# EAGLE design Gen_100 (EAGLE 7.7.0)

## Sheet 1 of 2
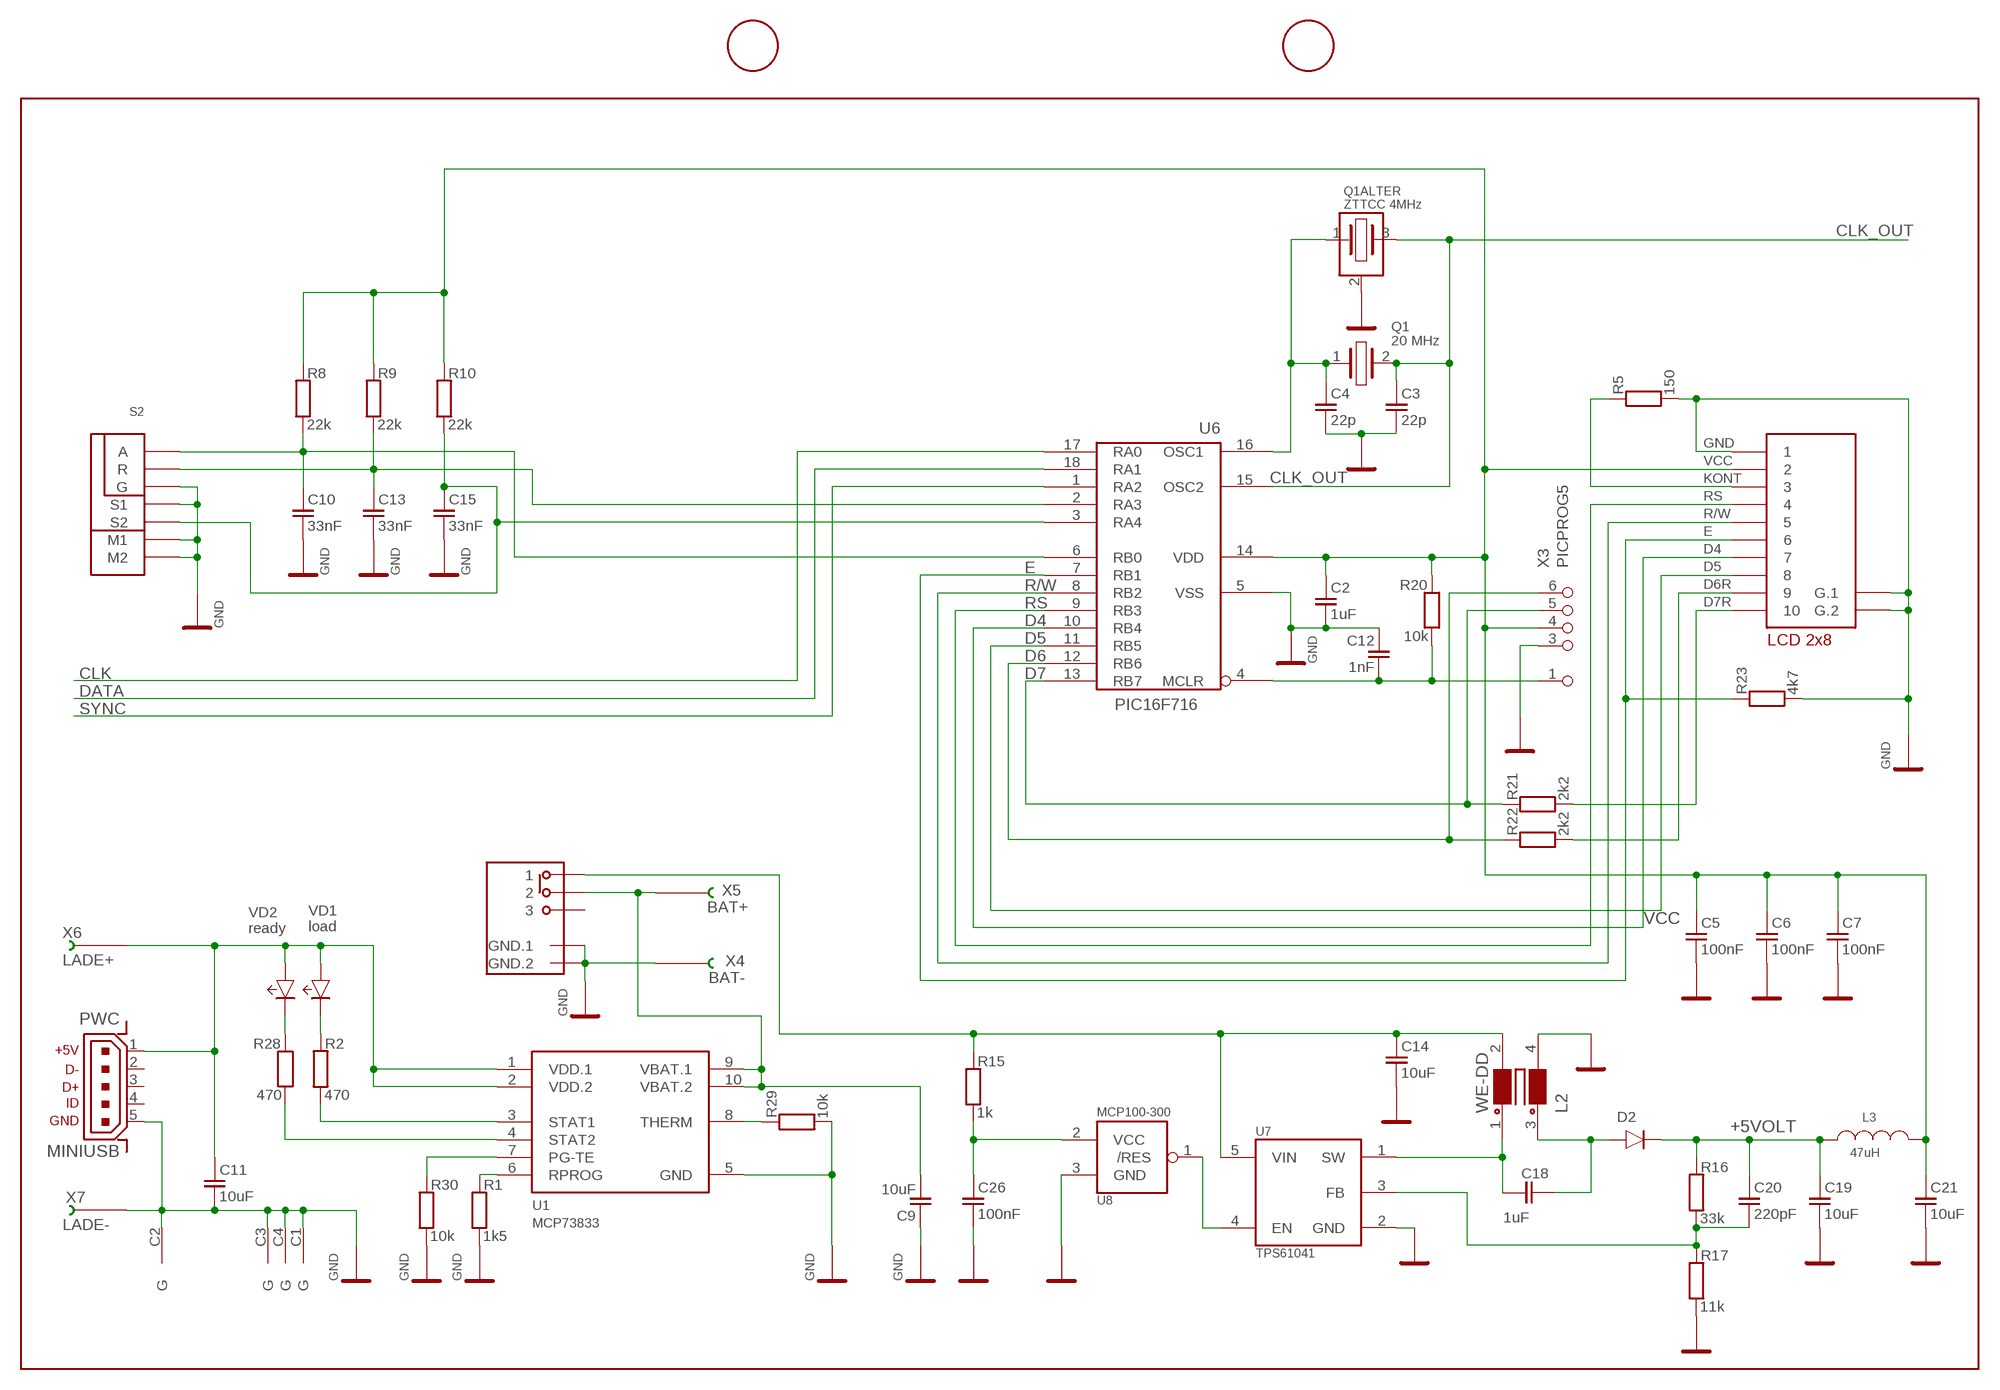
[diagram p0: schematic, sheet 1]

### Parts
C2  1uF  SMD-0603  [SOT-0603]
C3  22p  SMD-0603  [SOT-0603]
C4  22p  SMD-0603  [SOT-0603]
C5  100nF  SMD-0603  [SOT-0603]
C6  100nF  SMD-0603  [SOT-0603]
C7  100nF  SMD-0603  [SOT-0603]
C9  10uF  SMD-0805  [SOT-0805]
C10  33nF  SMD-0603  [SOT-0603]
C11  10uF  SMD-0805  [SOT-0805]
C12  1nF  SMD-0603  [SOT-0603]
C13  33nF  SMD-0603  [SOT-0603]
C14  10uF  SMD-0805  [SOT-0805]
C15  33nF  SMD-0603  [SOT-0603]
C18  1uF  SMD-0805  [SOT-0805]
C19  10uF  SMD-0805  [SOT-0805]
C20  220pF  SMD-0603  [SOT-0603]
C21  10uF  SMD-0805  [SOT-0805]
C26  100nF  SMD-0603  [SOT-0603]
D2  BAR-43  [SOT-23]
L2  WE-DD  [WE-DD_7X7]
L3  47uH  SMD-1210  [SMD-1210]
PW  MINIUSB  [UX60A-MB-5SY]
Q1  20 MHz  Q-MA306  [Q-MA306]
Q1ALTER  ZTTCC 4MHz  ZTTCC  [ZTTCC]
R1  1k5  SMD-0603  [SMD-0603]
R2  470  SMD-0603  [SMD-0603]
R5  150  SMD-0603  [SMD-0603]
R8  22k  SMD-0603  [SMD-0603]
R9  22k  SMD-0603  [SMD-0603]
R10  22k  SMD-0603  [SMD-0603]
R15  1k  SMD-0603  [SMD-0603]
R16  33k  SMD-0603  [SMD-0603]
R17  11k  SMD-0603  [SMD-0603]
R20  10k  SMD-0603  [SMD-0603]
R21  2k2  SMD-0603  [SMD-0603]
R22  2k2  SMD-0603  [SMD-0603]
R23  4k7  SMD-0603  [SMD-0603]
R28  470  SMD-0603  [SMD-0603]
R29  10k  SMD-0603  [SMD-0603]
R30  10k  SMD-0603  [SMD-0603]
S1  FAR120-1431  SXUM-1X3  [SXUM1X3]
S2  DREHGEBER-ALPS5  [DG-ALPS-ST5]
U1  MCP73833  [MSOP10-0.5]
U6  PIC16F716  PIC16F627  [SO-18L]
U7  TPS61041  [SOT23-5]
U8  MCP100-300  TC1275  [SOT23]
VD1  load  LED-SMD  [LED0805]
VD2  ready  LED-SMD  [LED0805]
X2  FP10-1UPPE  [FPC10-1U]
X3  PICPROG5  [PICPROG5]
X4  BAT-  LÖTÖSEQ  [LÖTÖSEQ]
X5  BAT+  LÖTÖSEQ  [LÖTÖSEQ]
X6  LADE+  LÖTÖSEQ  [LÖTÖSEQ]
X7  LADE-  LÖTÖSEQ  [LÖTÖSEQ]

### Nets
+5VOLT: C19.2 C20.2 D2.3(K) L3.1 R16.2
CLK: U6.17(RA0) ; also sheet 2
CLK_OUT: C3.2 Q1.2 Q1ALTER.3 U6.15(OSC2) ; also sheet 2
D4: U6.10(RB4) X2.7
D5: U6.11(RB5) X2.8
D6: R22.2 U6.12(RB6) X3.6
D6R: R22.1 X2.9
D7: R21.2 U6.13(RB7) X3.5
D7R: R21.1 X2.10
DATA: U6.18(RA1) ; also sheet 2
E: R23.2 U6.7(RB1) X2.6
GND: C2.1 C3.1 C4.1 C5.1 C6.1 C7.1 C9.2 C10.1 C11.1 C12.2 C13.1 C14.1 C15.1 C19.1 C21.1 C26.1 L2.4 PW.5 PW.C1(G) PW.C2(G) PW.C3(G) PW.C4(G) Q1ALTER.2 R1.1 R5.1 R17.1 R23.1 R29.1 R30.1 S1.GND.1 S1.GND.2 S2.G S2.M1 S2.M2 S2.S1 U1.5(GND) U6.5(VSS) U7.2(GND) U8.3(GND) X2.1 X2.P$1(G.1) X2.P$2(G.2) X3.3 X4.1 X7.1 ; also sheet 2
KONT: R5.2 X2.3
MCLR_VPP: C12.1 R20.1 U6.4(MCLR) X3.1
N$1: R2.2 VD1.K
N$2: C11.2 PW.1 U1.1(VDD.1) U1.2(VDD.2) VD1.A VD2.A X6.1
N$3: R28.2 VD2.K
N$5: C4.2 Q1.1 Q1ALTER.1 U6.16(OSC1)
N$7: R2.1 U1.3(STAT1)
N$8: R28.1 U1.4(STAT2)
N$9: C9.1 S1.2 U1.9(VBAT.1) U1.10(VBAT.2) X5.1
N$10: R30.2 U1.7(PG-TE)
N$11: R1.2 U1.6(RPROG)
N$12: R29.2 U1.8(THERM)
N$15: U7.4(EN) U8.1(/RES)
N$17: C26.2 R15.1 U8.2(VCC)
N$19: C14.2 L2.2 R15.2 S1.1 U7.5(VIN)
N$20: C18.2 L2.1 U7.1(SW)
N$22: C10.2 R8.1 S2.A U6.6(RB0)
N$23: C13.2 R9.1 S2.R U6.2(RA3)
N$24: C15.2 R10.1 S2.S2 U6.3(RA4)
N$25: C18.1 D2.1(A) L2.3
N$27: C20.1 R16.1 R17.2 U7.3(FB)
R/W: U6.8(RB2) X2.5
RS: U6.9(RB3) X2.4
SYNC: U6.1(RA2) ; also sheet 2
VCC: C2.2 C5.2 C6.2 C7.2 C21.2 L3.2 R8.2 R9.2 R10.2 R20.2 U6.14(VDD) X2.2 X3.4 ; also sheet 2
Unconnected: PW.2 PW.3 PW.4 S1.3

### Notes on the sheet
- LCD 2x8

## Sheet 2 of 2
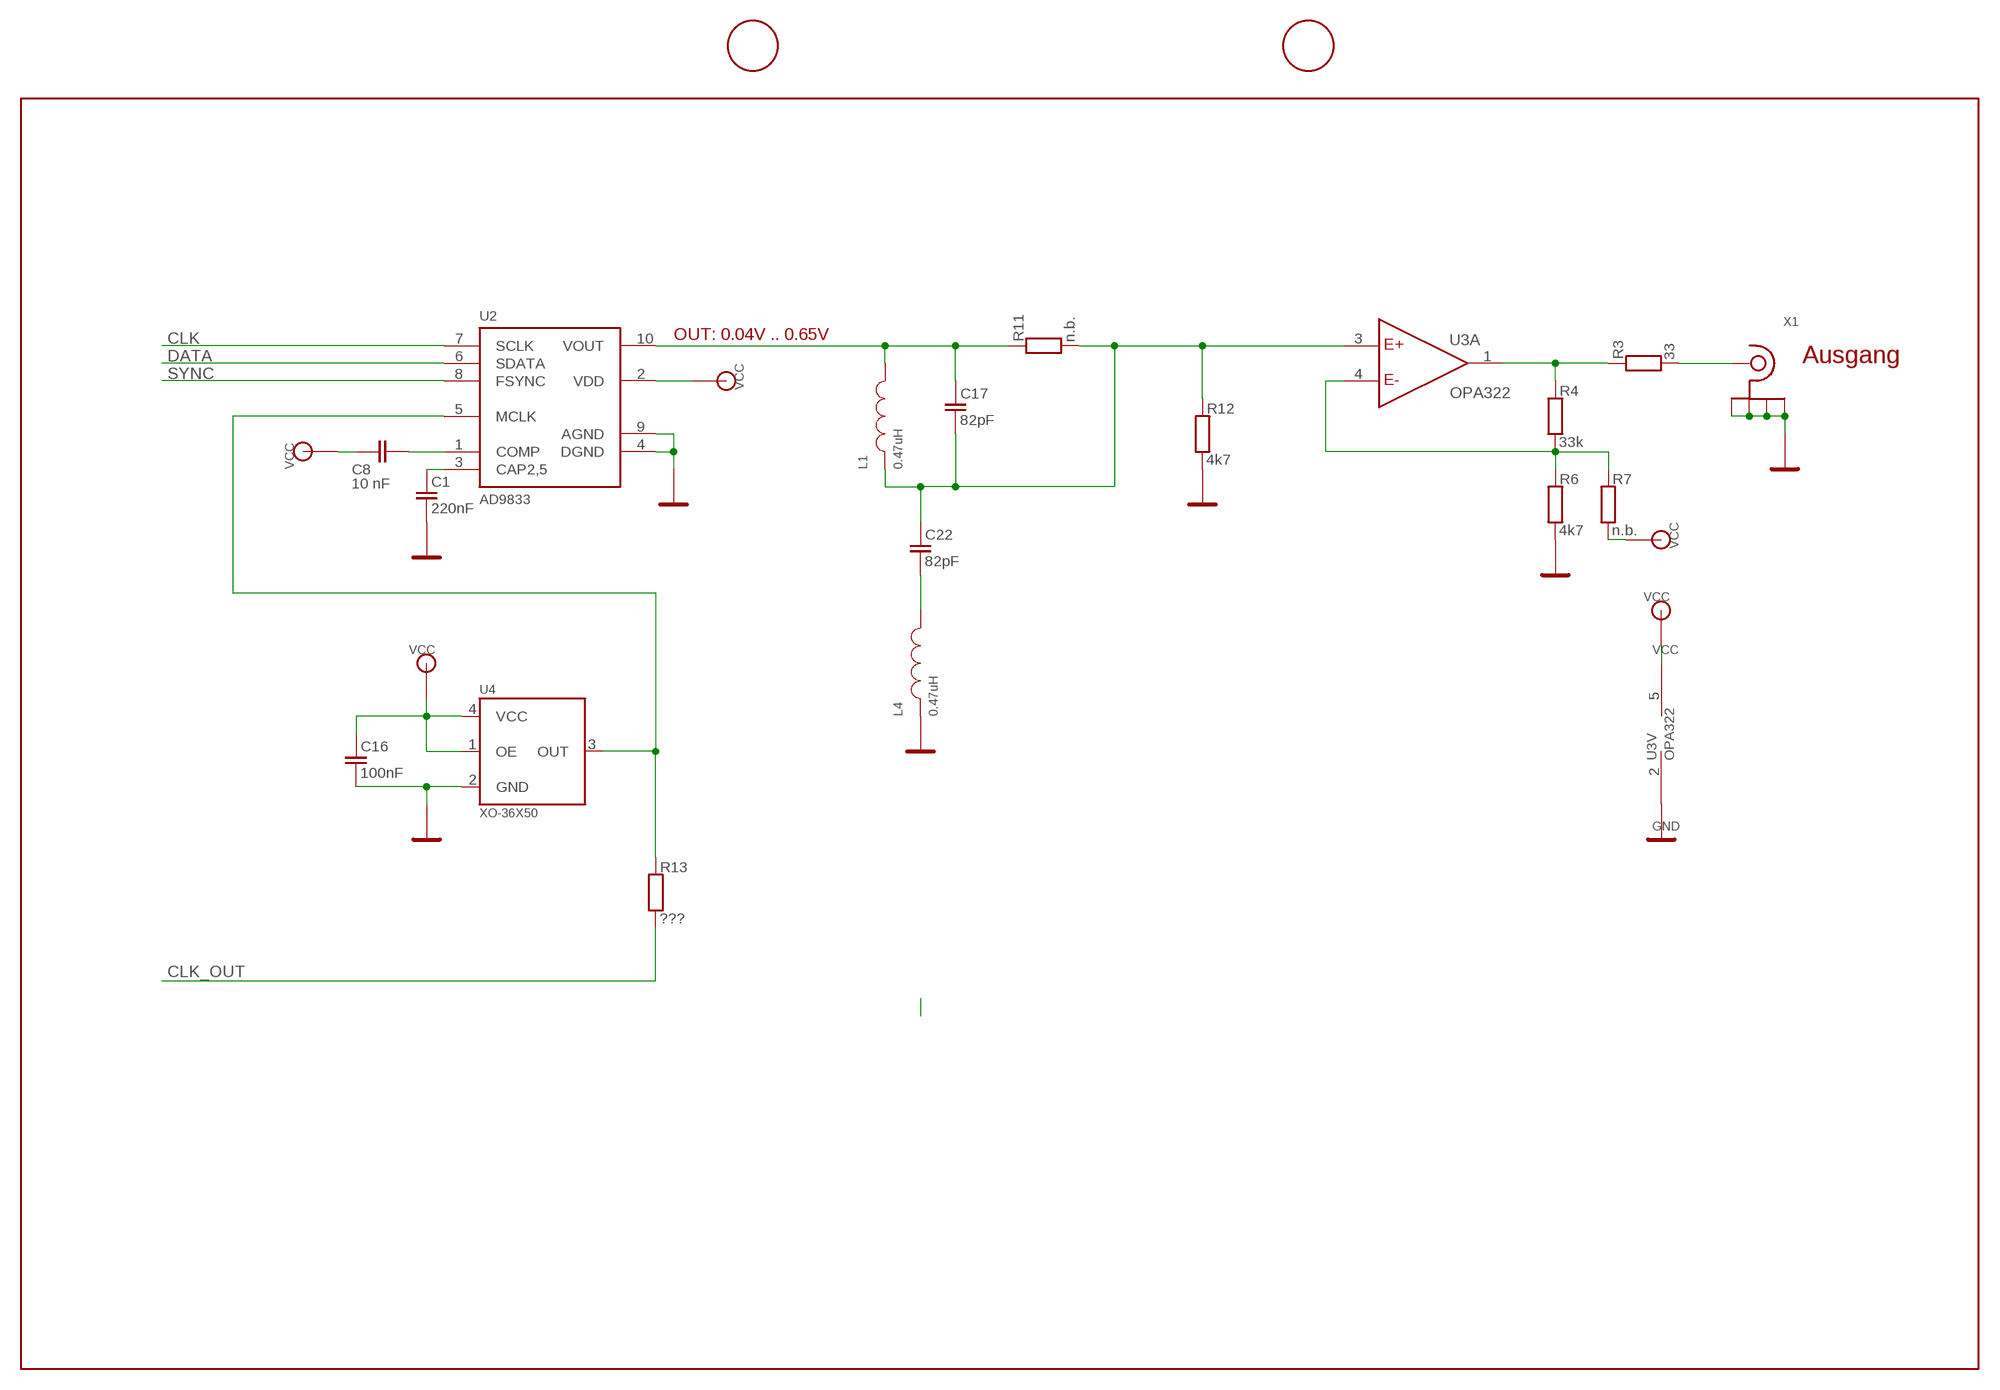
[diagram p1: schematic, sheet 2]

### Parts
C1  220nF  SMD-0603  [SOT-0603]
C8  10 nF  SMD-0603  [SOT-0603]
C16  100nF  SMD-0603  [SOT-0603]
C17  82pF  SMD-0603  [SOT-0603]
C22  82pF  SMD-0603  [SOT-0603]
L1  0.47uH  SMDL-0805  [SMDL-0805]
L4  0.47uH  SMDL-0805  [SMDL-0805]
R3  33  SMD-0805  [SMD-0805]
R4  33k  SMD-0603  [SMD-0603]
R6  4k7  SMD-0603  [SMD-0603]
R7  n.b.  SMD-0603  [SMD-0603]
R11  n.b.  SMD-0603  [SMD-0603]
R12  4k7  SMD-0603  [SMD-0603]
R13  ???  SMD-0603  [SMD-0603]
U2  AD9833  [RM-10]
U3  OPA322  [SOT23-5]
U4  XO-36X50  [XO-36X50]
X1  SMA-EDGE  [SMA-EDGE]

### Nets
CLK: U2.7(SCLK) ; also sheet 1
CLK_OUT: R13.1 ; also sheet 1
DATA: U2.6(SDATA) ; also sheet 1
GND: C1.1 C16.1 L4.1 R6.1 R12.1 U2.4(DGND) U2.9(AGND) U3.2(V:GND) U4.2(GND) X1.GND@1(GND) X1.GND@2(GND) X1.GND@3(GND) X1.GND@4(GND) ; also sheet 1
N$6: R3.2 R4.2 U3.1(A:O)
N$13: R3.1 X1.A
N$14: C17.2 L1.2 R11.2 U2.10(VOUT)
N$16: C1.2 U2.3(CAP2,5)
N$18: C8.1 U2.1(COMP)
N$21: R4.1 R6.2 R7.2 U3.4(A:E-)
N$28: R13.2 U2.5(MCLK) U4.3(OUT)
N$29: C17.1 C22.2 L1.1 R11.1 R12.2 U3.3(A:E+)
N$31: C22.1 L4.2
SYNC: U2.8(FSYNC) ; also sheet 1
VCC: C8.2 C16.2 R7.1 U2.2(VDD) U3.5(V:VCC) U4.1(OE) U4.4(VCC) ; also sheet 1

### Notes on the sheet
- OUT: 0.04V .. 0.65V
- Ausgang

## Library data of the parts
C1-C8 C10 C12 C13 C15-C17 C20 C22 C26 = C_KERAM:SMD-0603
C9 C11 C14 C18 C19 C21 = C_KERAM:SMD-0805
D2 = DIODEN:BAR-43
L1 L4 = L:SMDL-0805
L2 = L:WE-DD
L3 = L:SMD-1210
PW = mini-usb:MINIUSB
Q1 = Z_SPECIA:Q-MA306
Q1ALTER = Z_SPECIA:ZTTCC
R1 R2 R4-R13 R15-R17 R20-R23 R28-R30 = R:SMD-0603
R3 = R:SMD-0805
S1 = HAMRAD:SXUM-1X3
S2 = HAMRAD:DREHGEBER-ALPS5: Drehgeber von ALPS mit Taster, alle Wechsel zwischen den Rastunngen
U1 = MIC_CHIP:MCP73833
U2 = ANALOG_D:AD9833
U3 = TI_OPV:OPA322
U4 = Z_SPECIA:XO-36X50: MEMS Oszillator, programmierbar, 5x3.6
U6 = MIC_CHIP:PIC16F627
U7 = TI:TPS61041
U8 = MIC_CHIP:TC1275
VD1 VD2 = DIODEN:LED-SMD
X1 = HAMRAD:SMA-EDGE
X2 = Z_CONNEC:FP10-1UPPE
X3 = PINHD-Q:PICPROG5
X4-X7 = Z_CONNEC:LÖTÖSEQ

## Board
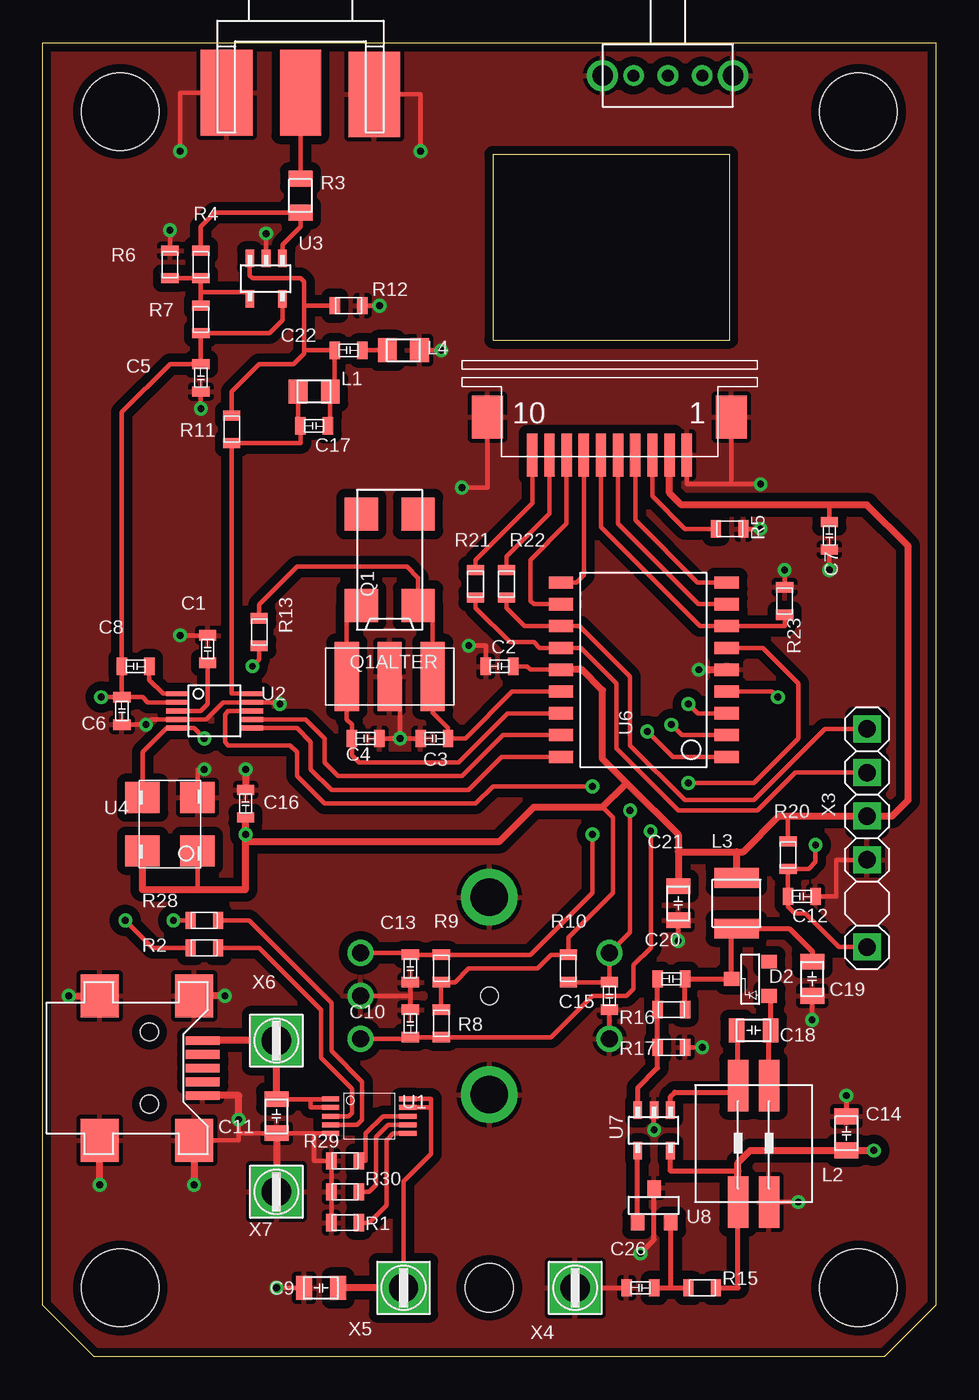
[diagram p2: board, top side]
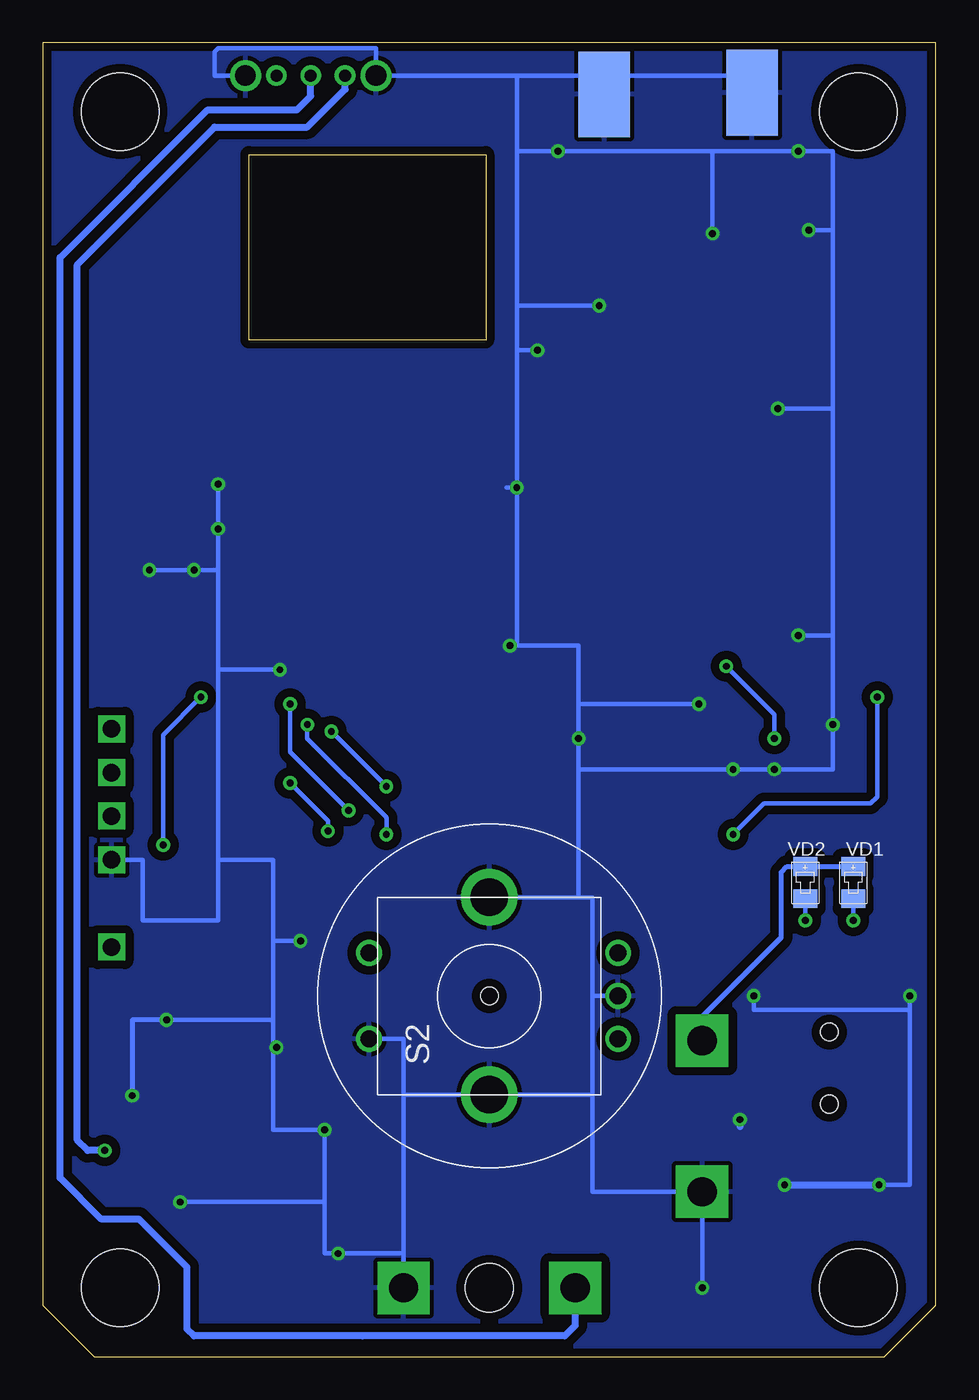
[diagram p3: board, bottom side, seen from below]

Size 52 x 76.5 mm. Coordinates in mm from the lower left corner, seen from the top.
Outline: 26.2,70 26.2,59.2 40,59.2 40,70 26.2,70
Copper layers (1*16): Top 0.035mm / dielectric 1.5mm / Bottom 0.035mm
Design rules "default *": minimum track width 0.15mm, minimum drill 0.3mm, track to track 0.15mm, track to pad 0.15mm, pad to pad 0.15mm, via to via 0.15mm, smd to smd 0mil, copper to edge 0.15mm, drill to drill 0.15mm, minimum pad ring 0.15mm, minimum via ring 0.15mm, stop-mask expansion 4mil, vias tented up to drill 0mil, thermal gap 10mil
Holes 2.8 mm at 26,4
Holes 1 mm at 26,21

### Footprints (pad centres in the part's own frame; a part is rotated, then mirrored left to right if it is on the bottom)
SOT-0603 = smd 0.6 x 1: 1 -0.8,0; 2 0.8,0
SOT-0805 = smd 0.914 x 1.397: 1 -0.991,0; 2 0.991,0
SOT-23 = smd 0.8 x 0.9: 1 -1,-1.1; 2 1,-1.1; 3 0,1.1
SMDL-0805 = smd 1.092 x 1.397: 1 -0.94,0; 2 0.94,0
WE-DD_7X7 = smd 1.2 x 3: 1 0.91,-3.39; 2 0.91,3.41; 3 -0.89,-3.39; 4 -0.89,3.41
SMD-1210 = smd 1.143 x 2.591: 1 -1.473,0; 2 1.473,0
UX60A-MB-5SY = smd 0.5 x 2: 1 -1.6,3.1; 2 -0.8,3.1; 3 0,3.1; 4 0.8,3.1; 5 1.6,3.1 | smd 2.5 x 2.2: C1 -4.2,2.6; C2 -4.2,-2.9; C3 4.2,-2.9; C4 4.2,2.6 | hole 1.016: -2.1,0; 2.1,0
Q-MA306 = smd 1.93 x 1.93: 1 -2.667,1.651; 2 -2.667,-1.651; 3 2.667,-1.651; 4 2.667,1.651
ZTTCC = smd 1.4 x 4: 1 -2.5,0; 2 0,0; 3 2.5,0
SMD-0603 = smd 0.6 x 1: 1 -0.8,0; 2 0.8,0
SMD-0805 = smd 0.914 x 1.397: 1 -0.991,0; 2 0.991,0
SXUM1X3 = drill 0.7 pad 1.2: 1 -2,0; 2 0,0; 3 2,0 | drill 1.2 pad 1.7: GND.1 -3.8,0; GND.2 3.8,0
DG-ALPS-ST5 = drill 1: A -2.5,-7.5; G 0,-7.5; R 2.5,-7.5; S1 -2.5,7; S2 2.5,7 | drill 2.2: M1 -5.75,0; M2 5.75,0
MSOP10-0.5 = smd 1 x 0.29: 1 -2.25,1; 2 -2.25,0.5; 3 -2.25,0; 4 -2.25,-0.5; 5 -2.25,-1; 6 2.25,-1; 7 2.25,-0.5; 8 2.25,0; 9 2.25,0.5; 10 2.25,1
RM-10 = smd 0.279 x 1.27: 1 -1,-2.2; 2 -0.5,-2.2; 3 0,-2.2; 4 0.5,-2.2; 5 1,-2.2; 6 1,2.2; 7 0.5,2.2; 8 0,2.2; 9 -0.5,2.2; 10 -1,2.2
SOT23-5 = smd 0.508 x 1.016: 1 -0.953,-1.143; 2 0,-1.143; 3 0.953,-1.143; 4 0.953,1.206; 5 -0.953,1.206
XO-36X50 = smd 1.8 x 2: 1 -1.55,-1.6; 2 1.55,-1.6; 3 1.55,1.6; 4 -1.55,1.6
SO-18L = smd 0.711 x 1.422: 1 -5.08,-4.826; 2 -3.81,-4.826; 3 -2.54,-4.826; 4 -1.27,-4.826; 5 0,-4.826; 6 1.27,-4.826; 7 2.54,-4.826; 8 3.81,-4.826; 9 5.08,-4.826; 10 5.08,4.826; 11 3.81,4.826; 12 2.54,4.826; 13 1.27,4.826; 14 0,4.826; 15 -1.27,4.826; 16 -2.54,4.826; 17 -3.81,4.826; 18 -5.08,4.826
SOT23-5' = smd 1.016 x 0.508: 1 -1.143,0.953; 2 -1.143,0; 3 -1.143,-0.953; 4 1.206,-0.953; 5 1.206,0.953
SOT23 = smd 0.889 x 0.787: 1 -1.016,0.965; 2 -1.016,-0.965; 3 1.016,0
ABS-100 = hole 4.5: -21.5,68.5; 21.5,68.5; -21.5,0; 21.5,0
LED0805 = smd 1.092 x 1.397: A 0.94,0; K -0.94,0
SMA-EDGE = smd 5 x 2.4: A 0,0 | smd 5 x 3: GND@1 0,4.3; GND@2 -0.1,-4.3 | smd 5 x 3 bottom: GND@3 0,4.3; GND@4 -0.1,-4.3
FPC10-1U = smd 0.6 x 2.5: 1 -4.5,1.5; 2 -3.5,1.5; 3 -2.5,1.5; 4 -1.5,1.5; 5 -0.5,1.5; 6 0.5,1.5; 7 1.5,1.5; 8 2.5,1.5; 9 3.5,1.5; 10 4.5,1.5 | smd 1.8 x 2.5: P$1 7.1,-0.7; P$2 -7.1,-0.7
PICPROG5 = drill 1.016 pad 1.575 square: 1 -6.35,0; 3 -1.27,0; 4 1.27,0; 5 3.81,0; 6 6.35,0
LÖTÖSEQ = drill 1.702 pad 3.048 square: 1 0,0

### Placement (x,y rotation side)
C1  9.6,41.2 270 top
C2  26.6,40.2 0 top
C3  22.8,36 0 top
C4  18.8,36 180 top
C5  9.2,57 90 top
C6  4.6,37.6 90 top
C7  45.8,47.8 90 top
C8  5.4,40.2 180 top
C9  16.2,4 180 top
C10  21.4,19.4 270 top
C11  13.6,14 90 top
C12  44.2,26.8 0 top
C13  21.4,22.6 90 top
C14  46.8,13 270 top
C15  33,21 90 top
C16  11.8,32.2 270 top
C17  15.8,54.2 180 top
C18  41.4,19 180 top
C19  44.8,22 90 top
C20  36.6,22 0 top
C21  37,26.4 90 top
C22  17.8,58.6 180 top
C26  34.8,4 0 top
D2  41.2,22 90 top
L1  15.8,56.2 180 top
L2  41.4,12.4 180 top
L3  40.4,26.4 90 top
L4  21,58.6 180 top
PW  6.2,16.8 270 top
Q1  20.2,46.4 90 top
Q1ALTER  20.2,39.6 0 top
R1  17.6,7.8 0 top
R2  9.4,23.8 180 top
R3  15,67.6 270 top
R4  9.2,63.6 90 top
R5  40,48.2 180 top
R6  7.4,63.6 270 top
R7  9.2,60.4 90 top
R8  23.2,19.4 90 top
R9  23.2,22.6 270 top
R10  30.6,22.6 90 top
R11  11,54 270 top
R12  17.8,61.2 180 top
R13  12.6,42.2 270 top
R15  38.4,4 0 top
R16  36.6,20.2 0 top
R17  36.6,18 180 top
R20  43.4,29.2 90 top
R21  25.2,45 270 top
R22  27,45 270 top
R23  43.2,44 270 top
R28  9.4,25.4 180 top
R29  17.6,11.4 0 top
R30  17.6,9.6 0 top
S1  36.4,74.6 0 top
S2  26,21 90 bottom
U1  19,14 0 top
U2  10,37.6 270 top
U3  13,62.8 180 top
U4  7.4,31 90 top
U6  35,40 90 top
U7  TPS61041  [SOT23-5']  35.6,13.2 270 top
U8  35.6,8.8 90 top
U$13  [ABS-100]  26,4 0 bottom
VD1  4.8,27.6 90 bottom
VD2  7.6,27.6 90 bottom
X1  15,73.6 90 top
X2  33,54 180 top
X3  48,30.2 90 top
X4  31,4 0 top
X5  21,4 0 top
X6  13.6,18.4 0 top
X7  13.6,9.6 0 top

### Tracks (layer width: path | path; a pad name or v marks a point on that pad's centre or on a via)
+5VOLT
  Top 0.3: 40.1,24.93 D2.3 C20.2 R16.2 | C19.2 44.8,23.6 43.47,24.93 L3.1
  Top 0.4: 40.1,24.93 L3.1
CLK
  Top 0.25: U6.17 26.79,36.19 24.4,33.8 17.2,33.8 16.4,34.6 16.4,36 15.3,37.1 U2.7
CLK_OUT
  Top 0.25: U6.15 27.33,38.73 24.6,36 C3.2 23.6,36.6 22.7,37.5 Q1ALTER.3 22.7,43.73 Q1.2 21.85,45.35 21.2,46 14.8,46 12.6,43.8 R13.1
D4
  Top 0.25: X2.7 31.5,45.5 31.08,45.08 U6.10
D5
  Top 0.25: X2.8 30.5,48.5 28.4,46.4 28.4,44 28.59,43.81 U6.11
D6
  Top 0.25: X3.6 45.55,36.55 41.4,32.4 37.4,32.4 34.2,35.6 34.2,36.6 34.2,39.6 31.26,42.54 U6.12 28.06,42.54 27,43.6 R22.2
D6R
  Top 0.25: X2.9 29.5,49.1 27,46.6 R22.1
D7
  Top 0.25: X3.5 43.81,34.01 41.6,31.8 37,31.8 33.4,35.4 33.4,37.2 33.4,38.6 33.4,39.2 31.33,41.27 U6.13 28.93,41.27 28.6,41.6 27.2,41.6 25.2,43.6 R21.2
D7R
  Top 0.25: X2.10 28.5,49.7 25.2,46.4 R21.1
DATA
  Top 0.25: U6.18 26.72,34.92 24.8,33 16.8,33 15.6,34.2 15.6,35.8 14.8,36.6 U2.6
E
  Top 0.25: X2.6 32.5,48.3 38.26,42.54 U6.7 43.2,42.54 R23.2
GND  (via drill 0.4 pad 0.8)
  Top 0.25: X2.P$1 25.9,50.6 v24.4,50.6 | 40.1,50.8 X2.P$2 | v41.8,50.8 40.1,50.8 | U1.5 15.8,13.01 | 15.8,13.01 C11.1 11.4,13.01 | 11.4,13.01 v11.4,13.8 | PW.C4 11.4,12.6 11.4,13.01 | v13.6,4 C9.2 | 15.8,13.01 15.8,11.4 R29.1 R30.1 R1.1 | L2.4 v44,9 | v37,24.2 C21.1 | v38.4,18 R17.1 | 21.4,21 C13.1 | S2.G 21.4,21 | 21.4,21 C10.1 | X2.1 37.5,50.8 40.1,50.8 | C12.2 46.2,26.8 46.2,28.93 X3.3 | v41.8,48.2 R5.1 | C2.1 25.8,41.4 v24.8,41.4 | v43.2,45.8 R23.1 | S2.S1 C15.1 | v13.8,38 13.7,38.1 U2.9 10.5,38.1 9.5,37.1 U2.4 6.3,37.1 v6,36.8 C6.1 | U4.2 9,34.2 v9.4,34.2 | v8,42 C1.1 | v45.8,45.8 C7.1 | X1.GND@3 8,73.6 v8,70.2 | v13,65.4 U3.2 | v7.4,65.6 R6.1 | v9.2,55.2 C5.1 | v19.6,61.2 R12.1 | v23.2,58.6 L4.1 | v20.8,36 C3.1 | v20.8,36 C4.1 | Q1ALTER.2 20.8,39.6 v20.8,36 | X1.GND@4 22,73.5 v22,70.2
  Top 0.3: X4.1 C26.1 | U8.3 35.6,6.8 v34.8,6 | v35.6,13.2 U7.2 | v44.8,19.6 C19.1 | v46.8,15.2 C14.1
  Top 0.4: C11.1 X7.1 | v3.3,10 PW.C3 | PW.C4 v8.8,10 | PW.5 11.4,15.2 v11.4,13.8 | v1.5,21 PW.C2 | v10.6,21 PW.C1 | v38.2,40 U6.5 | v11.8,34.2 C16.1
  Bottom 0.25: v24.4,50.6 25,50.6 | v13.6,4 X7.1 20,9.6 20,15.25 | 31,6 v34.8,6 35.6,6 35.6,9 | 31,6 X4.1 | 35.6,9 v35.6,13.2 38.6,13.2 38.6,18 | 35.6,9 v44,9 | 31,15.25 S2.M1 20,15.25 | 31,15.25 31,6 | 38.6,24.2 v37,24.2 | 38.6,18 38.6,19.6 | 38.6,19.6 38.6,24.2 | 38.6,19.6 v44.8,19.6 | 41.8,28.93 41.8,25.4 46.2,25.4 46.2,28.93 X3.3 | 38.6,24.2 38.6,28.93 41.8,28.93 | 38.6,18 v38.4,18 | 20,15.25 20,21 | 20,21 S2.G | 20.8,26.75 20,26.75 20,21 | 20.8,26.75 S2.M2 | 20.8,26.75 20.8,34.2 | 41.8,28.93 41.8,40 | v41.8,50.8 v41.8,48.2 41.8,45.8 | 41.8,40 v38.2,40 | 41.8,40 41.8,45.8 | v24.4,50.6 24.4,41.4 v24.8,41.4 20.8,41.4 20.8,38 | 41.8,45.8 v43.2,45.8 v45.8,45.8 | S2.S1 31,18.5 31,15.25 | 20.8,34.2 v20.8,36 20.8,38 | 20.8,38 v13.8,38 | 20.8,34.2 v11.8,34.2 v9.4,34.2 6,34.2 v6,36.8 6,42 | 6,42 v8,42 | X1.GND@3 10.7,74.6 19.3,74.6 | v24.4,50.6 24.4,57 | 24.4,61.2 24.4,58.6 | 24.4,70.2 24.4,61.2 | 6,42 6,55.2 | 6,55.2 6,65.6 | 6,65.6 6,70.2 v8,70.2 13,70.2 | 13,70.2 v22,70.2 24.4,70.2 | 20.4,74.6 19.3,74.6 | 19.3,74.6 X1.GND@4 20.4,74.6 | 13,70.2 v13,65.4 | 6,65.6 v7.4,65.6 | 6,55.2 v9.2,55.2 | S1.GND.2 42,74.6 42,76 41.8,76.2 32.6,76.2 S1.GND.1 24.4,74.6 | 1.5,20.2 v1.5,21 | 1.5,20.2 10.6,20.2 v10.6,21 | v3.3,10 1.5,10 1.5,20.2 | 24.4,61.2 v19.6,61.2 | 24.4,58.6 24.4,47.4 | 24.4,58.6 v23.2,58.6 | 24.4,74.6 20.4,74.6 | 24.4,70.2 24.4,74.6
  Bottom 0.3: v46.8,15.2 46.8,19.6 v44.8,19.6
  Bottom 0.4: v8.8,10 v3.3,10 | v11.4,13.8 11.4,13.4
  pour Bottom (isolate 0.5): 0.4,76 0.4,3 3,0.4 49,0.4 51.6,3 51.6,76
  pour Top (isolate 0.5): 0.6,76 0.4,3.4 3.4,0.4 48.8,0.4 51.6,3.2 51.6,76.2
KONT
  Top 0.25: X2.3 35.5,50.1 37.4,48.2 R5.2
MCLR_VPP  (via drill 0.4 pad 0.8)
  Top 0.25: U6.4 42.47,38.73 v42.8,38.4 | v45,29.8 45,28.8 44.6,28.4 R20.1 C12.1 43.4,26.2 43.8,25.8 44.4,25.8 46.35,23.85 X3.1
  Bottom 0.25: v45,29.8 45,35.2 45,36.2 v42.8,38.4
N$1  (via drill 0.4 pad 0.8)
  Top 0.25: v4.8,25.4 6.4,23.8 R2.2
  Bottom 0.25: VD1.K v4.8,25.4
N$2
  Top 0.25: C11.2 15.6,14.99 | 15.6,14.99 U1.1 | U1.2 15.6,14.5 15.6,14.99
  Top 0.4: PW.1 X6.1 C11.2
  Bottom 0.3: VD1.A VD2.A 8.66,28.54 9,28.2 9,24.4 13.6,19.8 13.6,19.2 X6.1
N$3  (via drill 0.4 pad 0.8)
  Top 0.25: v7.6,25.4 R28.2
  Bottom 0.25: VD2.K v7.6,25.4
N$5
  Top 0.25: U6.16 27.06,37.46 24.2,34.6 18.4,34.6 18,35 C4.2 18,36.8 17.7,37.1 Q1ALTER.1 17.7,43.73 Q1.1
N$6
  Top 0.25: U3.1 13.95,64.75 15,65.8 R3.2 10.01,66.61 9.2,65.8 R4.2
N$7
  Top 0.25: U1.3 17.8,14 18,14.2 18,15.6 16.2,17.4 16.2,20.2 12.6,23.8 R2.1
N$8
  Top 0.25: U1.4 18.3,13.5 18.6,13.8 18.6,16 16.8,17.8 16.8,20.6 12,25.4 R28.1
N$9
  Top 0.25: X5.1 21,10.2 22.6,11.8 22.6,14.4 | 22.6,14.4 22.6,15 U1.10 | U1.9 22.5,14.5 22.6,14.4
  Top 0.4: X5.1 C9.1
  Bottom 0.4: S1.2 36.4,73.4 37.2,72.6 42.4,72.6 51,64 51,10.4 48.6,8 46.4,8 43.6,5.2 43.6,1.6 43.2,1.2 33.4,1.2 21.6,1.2 21,1.8 X5.1
N$10
  Top 0.25: U1.7 20.1,13.5 19.4,12.8 19.4,10 19,9.6 R30.2
N$11
  Top 0.25: U1.6 20.4,13 20,12.6 20,8.8 19,7.8 R1.2
N$12
  Top 0.25: U1.8 19.8,14 18.8,13 18.8,11.4 R29.2
N$13
  Top 0.25: R3.1 X1.A
N$14
  Top 0.25: U2.10 11,38.6 R11.2 15,53.2 C17.2 14.86,54.2 L1.2
N$15
  Top 0.3: U8.1 34.63,11.99
  Top 0.4: 34.63,11.99 U7.4
N$16
  Top 0.25: U2.3 9.2,37.6 9.6,38 C1.2
N$17
  Top 0.3: 36.56,4 U8.2 | C26.2 36.56,4 | 36.56,4 R15.1
N$18
  Top 0.25: U2.1 7,38.6 6.2,39.4 C8.1
N$19  (via drill 0.4 pad 0.8)
  Top 0.3: U7.5 36.55,10.8 40.49,10.8 | C14.2 | L2.2 40.49,4 R15.2
  Top 0.4: v48.4,12 C14.2 41.2,12 40.49,11.29 40.49,10.8 L2.2
  Bottom 0.4: S1.1 34.4,73.8 36.6,71.6 42,71.6 50,63.6 50,12.6 49.4,12 v48.4,12
N$20
  Top 0.3: C18.2 40.49,19 L2.1 40.49,15.4 36.8,15.4 36.55,15.15 U7.1
N$21
  Top 0.25: R6.2 R4.1 9.2,62 | U3.4 12.05,62 9.2,62 | R7.2 9.2,62
N$22  (via drill 0.4 pad 0.8)
  Top 0.25: S2.A 21.4,18.5 C10.2 R8.1 29.6,18.6 32,21 34,21 34.4,21.4 34.4,22.8 35.4,23.8 v35.4,30.6 | U6.6 41.93,41.27 44,39.2 44,36 41.4,33.4 v37.6,33.4
  Bottom 0.25: v37.6,33.4 35.4,31.2 v35.4,30.6
N$23  (via drill 0.4 pad 0.8)
  Top 0.25: S2.R 21.4,23.5 C13.2 R9.1 28.4,23.4 32,27 v32,30.4 | U6.2 37.21,36.19 v36.6,36.8
  Bottom 0.25: v36.6,36.8 36.6,36 32,31.4 32,31 v32,30.4
N$24  (via drill 0.4 pad 0.8)
  Top 0.25: U6.3 38.14,37.46 v37.6,38 | v34.2,31.8 34.2,24.7 S2.S2 C15.2 R10.1
  Bottom 0.25: v37.6,38 37.6,35.2 v34.2,31.8
N$25
  Top 0.3: 42.39,21 C18.1 42.29,19 L2.3
  Top 0.4: 42.39,21 D2.1
N$27
  Top 0.3: C20.1 R16.1 R17.2 35.8,16.8 34.65,15.65 U7.3
N$28  (via drill 0.4 pad 0.8)
  Top 0.25: U4.3 5.8,35.2 7.2,36.6 U2.5 8.8,36.6 v9.4,36 | v12.2,40.2 12.6,40.6 R13.2
  Bottom 0.25: v9.4,36 9.4,37.4 v12.2,40.2
N$29
  Top 0.25: U3.3 12.05,62.95 12.2,62.8 15,62.8 15.2,62.6 15.2,61.2 | 15.2,58.6 15.2,58.4 14.6,57.8 12.6,57.8 11,56.2 R11.1 | 15.2,58.6 15.2,61.2 | 15.2,61.2 R12.2 | 15.2,58.6 C22.2 17,56.2 L1.1 16.74,54.2 C17.1
N$31
  Top 0.25: L4.2 C22.1
R/W
  Top 0.25: X2.5 33.5,48.5 38.19,43.81 U6.8
RS
  Top 0.25: X2.4 34.5,48.7 38.12,45.08 U6.9
SYNC  (via drill 0.4 pad 0.8)
  Top 0.25: U6.1 36.68,34.92 v35.2,36.4 | v32,33.2 26.2,33.2 25.2,32.2 16.4,32.2 14.8,33.8 14.8,35.2 14.4,35.6 10.8,35.6 10.6,35.8 10.6,37.4 10.8,37.6 U2.8
  Bottom 0.25: v32,33.2 v35.2,36.4
VCC  (via drill 0.4 pad 0.8)
  Top 0.25: R8.2 R9.2 24,21.8 24.8,22.6 28.8,22.6 29.6,23.4 R10.2 30.6,24.4 33.2,27 33.2,31.4 32.6,32 | 43.4,31.47 R20.2 | U6.14 28.4,40 28.2,40.2 C2.2 | 33.9,33.3 34.1,33.3 | 9,27.2 U4.1 | v3.4,38.4 C6.2 | 11.8,29.8 v11.8,30.4 | U2.2 6.1,38.1 5.8,38.4 C6.2 | C6.2 C8.2 4.6,55 7.4,57.8 C5.2 R7.1 13.2,59.6 13.95,60.35 U3.5 | 45.8,49.6 C7.2
  Top 0.4: 40.4,29.4 L3.2 | 40.4,29.4 40.8,29.4 42.87,31.47 43.4,31.47 X3.4 49.47,31.47 50.4,32.4 50.4,47.2 48,49.6 45.8,49.6 37.2,49.6 36.5,50.3 X2.2 | 37,29.4 C21.2 | 37,29.4 40.4,29.4 | U6.14 31.4,40 32.6,38.8 32.6,34.8 34.1,33.3 37,30.4 37,29.4 | 33.9,33.3 32.6,32 28.6,32 26.6,30 11.8,30 | U4.4 5.8,27.2 9,27.2 11.8,27.2 11.8,29.8 11.8,30 | 11.8,30 v11.8,30.4 C16.2
  Bottom 0.25: v3.4,38.4 3.4,32.6 3.8,32.2 10,32.2 v11.8,30.4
